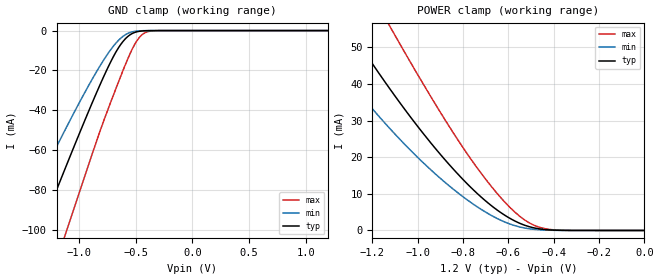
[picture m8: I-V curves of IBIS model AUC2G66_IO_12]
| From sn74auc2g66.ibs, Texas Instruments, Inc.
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[Model]   AUC2G66_IO_12
Model_type  Terminator
| variable   typ   min   max
C_comp   3.76pF   3.34pF   3.91pF
| C_tri-state   3.76pF   3.34pF   3.91pF
[Temperature Range]   40   100   -40
| Ambient temperature   25   85   -40
[Voltage range]   1.2   1.1   1.3
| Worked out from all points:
|   GND clamp passes 1 mA (typ) near -0.51 V on its own axis
|   POWER clamp passes 1 mA (typ) near -0.51 V on its own axis
[GND Clamp]
| AUC2G66_IO_12
|   Voltage   I(typ)   I(min)   I(max)
-2.7V     -295.9mA   -240.2mA   -365.2mA
-1.56V    -131.6mA   -100.3mA   -176.2mA
-1.36V    -102.8mA   -76.67mA   -142.5mA
-1.325V   -97.76mA   -72.6mA    -136.6mA
-1.125V   -69.29mA   -49.85mA   -102.6mA
-1.095V   -65.07mA   -46.53mA   -97.51mA
-755mV    -19.55mA   -12.26mA   -40.86mA
-655mV    -8.8mA     -5.013mA   -26.02mA
-570mV    -2.929mA   -1.401mA   -14.04mA
-470mV    -370uA     -148.5uA   -3.538mA
-365mV    -20.46uA   -9.75uA    -222.7uA
1.2V      342.3pA    8.238nA    218.2pA
[POWER Clamp]
| AUC2G66_IO_12
|   Voltage   I(typ)   I(min)   I(max)
-2.7V     211.1mA    181.9mA    241.3mA
-1.48V    72.52mA    55.24mA    96.17mA
-1.31V    55.75mA    41.41mA    76.64mA
-1.285V   53.38mA    39.49mA    73.8mA
-1.125V   38.83mA    27.95mA    55.96mA
-1.105V   37.1mA     26.61mA    53.78mA
-940mV    23.72mA    16.42mA    36.29mA
-795mV    13.58mA    8.96mA     22.12mA
-650mV    5.596mA    3.28mA     10.13mA
-545mV    1.833mA    886.2uA    3.634mA
-420mV    160.1uA    72.28uA    303uA
-35.59fV  342.3pA    660.1pA    251.8pA
